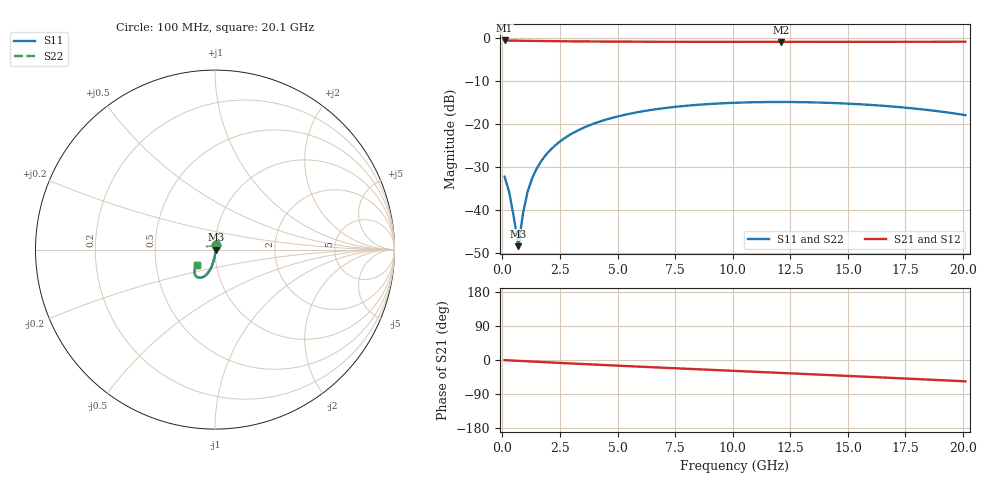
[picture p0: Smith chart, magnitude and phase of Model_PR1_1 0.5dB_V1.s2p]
!version-1
!date-07.2020
!Series
#	GHZ S RI R 50.0
!	FREQ.GHZ	S11RE	S11IM	S21RE	S21IM	S12RE	S12IM	S22RE	S22IM
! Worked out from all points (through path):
!   101 points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, 100 MHz to 20.1 GHz, reference 50 ohm
!   highest |S21| = -0.46 dB at 100 MHz (marker M1); lowest = -0.8 dB at 12.1 GHz (marker M2)
!   group delay of S21, straight-line fit = 7.65 ps
!   lowest |S11| = -48.3 dB at 700 MHz (marker M3), VSWR 1.01, Z = 50.4 - j0.11 ohm
!   |S11| at or under -10 dB: start of sweep to end of sweep
!   |S22| runs from -48.3 to -14.8 dB; largest |S21 - S12| = 0
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0.1  0.00605 0.0239  0.9489 -0.00632  0.9489 -0.00632  0.00605 0.0239
0.3  0.00536 0.0153  0.9466 -0.0166  0.9466 -0.0166  0.00536 0.0153
0.5  0.00457 0.00699  0.9444 -0.0267  0.9444 -0.0267  0.00457 0.00699
0.7  0.00368 -0.00109  0.9422 -0.0368  0.9422 -0.0368  0.00368 -0.00109
0.9  0.00269 -0.00892  0.9399 -0.0468  0.9399 -0.0468  0.00269 -0.00892
1.1  0.00162 -0.0165  0.9376 -0.0568  0.9376 -0.0568  0.00162 -0.0165
1.3  0.000458 -0.0238  0.9354 -0.0666  0.9354 -0.0666  0.000458 -0.0238
1.5  -0.000784 -0.0309  0.9331 -0.0764  0.9331 -0.0764  -0.000784 -0.0309
1.9  -0.0035 -0.0444  0.9284 -0.0957  0.9284 -0.0957  -0.0035 -0.0444
2.3  -0.0065 -0.0569  0.9237 -0.1147  0.9237 -0.1147  -0.0065 -0.0569
2.9  -0.0115 -0.074  0.9165 -0.1427  0.9165 -0.1427  -0.0115 -0.074
3.5  -0.0169 -0.0892  0.909 -0.1701  0.909 -0.1701  -0.0169 -0.0892
4.1  -0.0228 -0.1026  0.9012 -0.1969  0.9012 -0.1969  -0.0228 -0.1026
4.9  -0.031 -0.1178  0.8904 -0.2319  0.8904 -0.2319  -0.031 -0.1178
6.9  -0.0528 -0.1439  0.8604 -0.3157  0.8604 -0.3157  -0.0528 -0.1439
8.5  -0.0699 -0.1542  0.8328 -0.3793  0.8328 -0.3793  -0.0699 -0.1542
10.1  -0.0855 -0.157  0.8015 -0.4403  0.8015 -0.4403  -0.0855 -0.157
12.1  -0.1012 -0.1519  0.7567 -0.5131  0.7567 -0.5131  -0.1012 -0.1519
13.5  -0.1089 -0.144  0.7214 -0.5618  0.7214 -0.5618  -0.1089 -0.144
16.9  -0.1136 -0.1154  0.6213 -0.6723  0.6213 -0.6723  -0.1136 -0.1154
18.5  -0.1082 -0.0995  0.5673 -0.7198  0.5673 -0.7198  -0.1082 -0.0995
20.1  -0.0977 -0.0832  0.509 -0.7641  0.509 -0.7641  -0.0977 -0.0832
